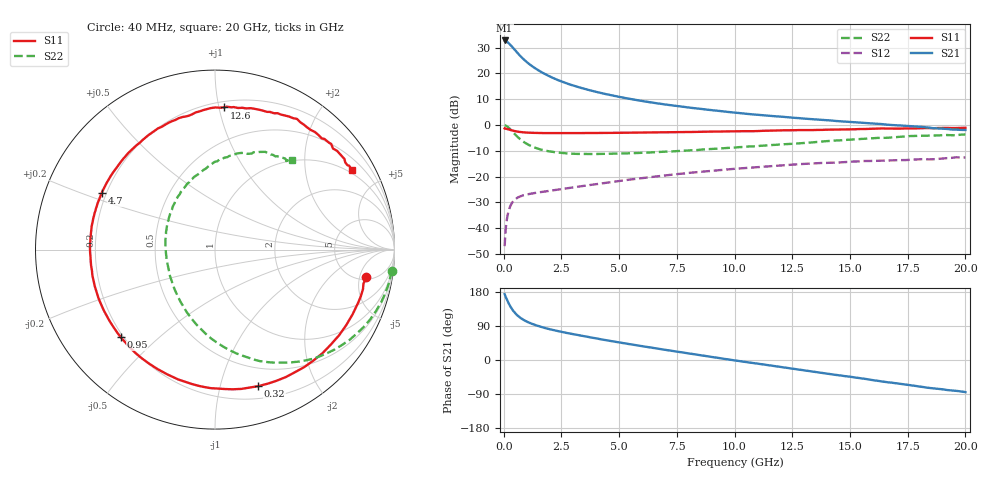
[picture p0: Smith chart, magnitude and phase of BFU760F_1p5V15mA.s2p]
! Filename:  P:\Prog\Test\Noise\ATS_data\Testdata_Net\Split files Spar\BFU760F_2W_C1_Bias4_1.5V_5mA_60mA_D.s2p
! Date/Time: Mon 06/Feb/2012 15:07:21
! BFU760_2W_C1_Bias4_1.5V_5mA_60mA_R.s2p
! MDIF S-parameter v. bias file
! BFU760_2W_C1_1.5V_5mA_60mA
! Date/time Fri Mar 18 11:09:37 2011
! VAR V_out= 1.5000
! VAR I_out= 15.0600
! VAR V_in= 0.7844
! VAR I_in= 0.0455
! Device data file deembeded for feedlines and parallel
! Original file: \Split files Spar\BFU760_2W_C1_Bias4_1.5V_5mA_60mA_R.s2p
! Feed-files: PR003V01_101208_Feed1.s2p, PR003V01_101208_Feed2.s2p
! Parallel-file: PR003V01_101208_Par.s2p
# MHz S MA R 50
!  Freq-MHz  S11-mag  S11-arg  S21-mag  S21-arg  S12-mag  S12-arg  S22-mag  S22-arg
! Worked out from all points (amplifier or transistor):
!   167 points, 40 MHz to 20 GHz, reference 50 ohm
!   highest |S21| = 32.8 dB at 40 MHz (marker M1)
!   |S21| within 3 dB of that: start of sweep to 418 MHz
!   unconditionally stable (mu >= 1): 4.724 GHz to 13.91 GHz
!   at 550 MHz: K = 0.19, MSG = 28.4 dB, |S12| = -28.5 dB
!   at 4.2 GHz: K = 0.96, MSG = 17.6 dB, |S12| = -22.7 dB
!   at 20 GHz: K = 0.89, MSG = 5.3 dB, |S12| = -12.6 dB
!   S11 on the Smith chart (normalised r, x): 40 MHz: 5.60, -6.36; 320 MHz: 0.31, -1.32; 950 MHz: 0.19, -0.38; 4.7 GHz: 0.18, +0.23; 12.6 GHz: 0.24, +1.03; 20 GHz: 0.88, +3.53
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40  0.8563 -10.2  43.65 174.0  0.004483 84.8  0.991 -6.8
50  0.8487 -12.9  43.55 172.0  0.005215 81.5  0.9885 -8.8
120  0.8436 -30.1  41.98 162.0  0.01299 75.3  0.9599 -20.9
180  0.8318 -44.0  40.02 154.1  0.01874 68.5  0.9178 -30.7
240  0.8153 -57.1  37.88 146.6  0.02359 62.6  0.8692 -39.7
320  0.7981 -72.4  34.62 138.2  0.02881 55.6  0.7982 -50.6
380  0.7844 -82.9  32.36 132.6  0.03189 51.5  0.7453 -57.6
460  0.7677 -94.7  29.41 126.2  0.03519 46.8  0.6838 -66.0
600  0.7442 -111.0  24.9 117.3  0.03907 40.8  0.59 -78.4
750  0.73 -124.1  21.14 110.2  0.04194 36.6  0.5162 -89.1
950  0.7172 -137.1  17.41 102.9  0.04455 33.3  0.4457 -100.8
1300  0.7053 -152.5  13.17 93.8  0.04781 30.5  0.372 -116.8
1850  0.698 -167.8  9.428 83.5  0.05207 29.5  0.316 -135.2
2500  0.6964 -179.7  7.003 74.3  0.05726 30.0  0.2893 -151.2
3400  0.699 167.9  5.182 63.6  0.06556 30.2  0.2757 -167.0
4700  0.7058 153.4  3.75 49.4  0.07913 29.4  0.2776 174.7
6800  0.7206 133.7  2.579 28.7  0.1031 23.8  0.301 151.8
10200  0.7595 105.4  1.708 -2.8  0.1439 8.2  0.373 120.8
12600  0.7937 86.5  1.379 -23.7  0.1718 -5.3  0.4353 101.3
13400  0.7993 80.8  1.295 -30.5  0.1805 -10.9  0.4622 95.1
16800  0.8542 54.7  1.002 -59.8  0.2065 -32.1  0.5733 69.1
20000  0.8829 30.0  0.8022 -84.8  0.2354 -53.5  0.6562 49.3
